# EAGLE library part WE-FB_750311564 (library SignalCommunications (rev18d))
WE-FB Flyback Transformer suitable for LT3573/ LT3574/ LT3575/ LT3748 Characteristics easy design in solution less external components needed small board space low cost no optocoupler needed! long term reliability voltage control no aging same external parts for different output voltages easy design of custom power supply due to standard circuit and change of transformers and two components for feedback loop Isolation voltage up to 2.5 kV Applications Isolated power design Sensor interfaces Isolated telecom converters Power over Ethernet Details see: http://katalog.we-online.de/en/pbs/WE-FB_Linear? Updated 2014-07-07 2014 (C) Wurth Elektronik
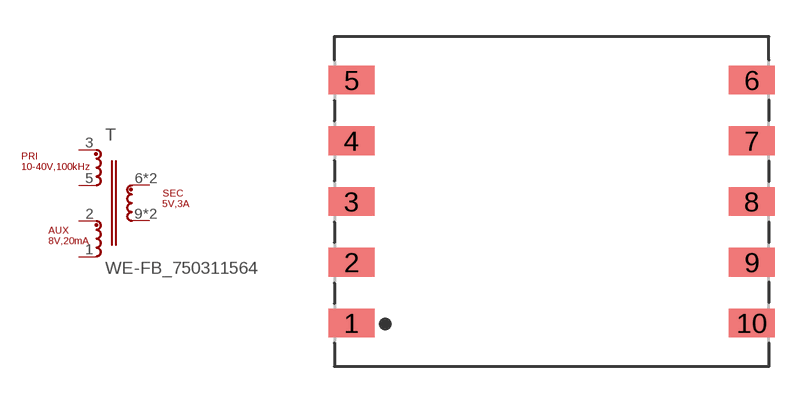
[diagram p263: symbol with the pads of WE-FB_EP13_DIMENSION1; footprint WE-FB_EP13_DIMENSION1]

Designator prefix T

## WE-FB_750311564  [WE-FB_EP13_DIMENSION1]
1  4  pas
2  5  pas
3  1  pas
5  6  pas
6  2  pas
7  2  pas
9  3  pas
10  3  pas

## Footprint WE-FB_EP13_DIMENSION1 (pad centres in mm)
smd 1.88 x 1.17: 1 -8.18,-4.96; 2 -8.18,-2.48; 3 -8.18,0; 4 -8.18,2.48; 5 -8.18,4.96; 6 8.18,4.96; 7 8.18,2.48; 8 8.18,0; 9 8.18,-2.48; 10 8.18,-4.96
